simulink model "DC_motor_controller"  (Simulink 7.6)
settings: Solver=ode14x  StartTime=0.0  StopTime=10  FixedStep=2e-5  RelTol=1e-3
InitFcn:
  | Ts=2e-5;
  | Kp=200;
  | Ki=300;
  | Acceler_max=250;
  | 
  | Kpi=10;
  | Kii=50;
StopFcn:
  | clc
  | close all
  | clear all
  | 
  | load Vit_Ia.mat
  | subplot 211
  | plot(x(1,:),x(3,:))
  | grid
  | axis([0 10 0 450])
  | title('courant Ia')
  | xlabel('temps')
  | 
  | subplot 212
  | plot(x(1,:),x(2,:),x(1,:),x(3,:))
  | title('Consigne et vitesse de rotation')
  | axis([0 10 0 450])
  | grid
  | xlabel('temps')
  | 
  | delete *.mat
undefined symbols (not defined in the file or in its folder): sigbuilder_block
libraries: powerlib x2, electricdrivelib x1

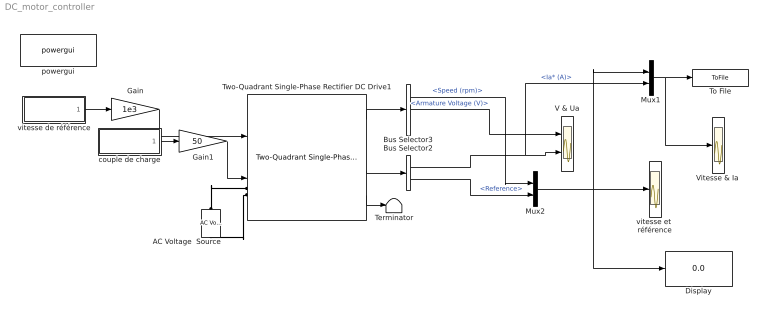
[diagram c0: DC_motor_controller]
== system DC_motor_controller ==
  AC Voltage  Source : powerlib/Electrical Sources/AC Voltage Source  DialogController=POWERSYS.PowerSysDialog  SystemSampleTime=-1  Amplitude=220  Phase=0  Frequency=60  SampleTime=0  Measurements=None
  Bus Selector2 : BusSelector  OutputSignals=Ia* (A),Reference
  Bus Selector3 : BusSelector  OutputSignals=Speed (rpm),Armature Voltage (V),Armature current ia (A)
  Display : Display
  Gain : Gain  Gain=1e3
  Gain1 : Gain  Gain=50
  Mux1 : Mux  Inputs=2
  Mux2 : Mux  Inputs=2
  Terminator : Terminator
  To File : ToFile  Filename=Vit_Ia  MatrixName=x
  Two-Quadrant Single-Phase Rectifier DC Drive1 : electricdrivelib/DC drives/Two-Quadrant Single-Phase Rectifier DC Drive  SystemSampleTime=-1  showMaskWarnings=on  AverageValue=off  MechanicalLoad=Torque Tm  driveType=DC1
  V & Ua : Scope  NumInputPorts=2
  "Vitesse & Ia " : Scope
  couple de charge : Subsystem  Tag=STV Subsys  LoadFcn=sigbuilder_block('load',[174.75 28.5 550.5 399.75 ]);  StartFcn=sigbuilder_block('start');  StopFcn=sigbuilder_block('stop');  ClipboardFcn=sigbuilder_block('clipboard');
  powergui : powerlib/powergui  Priority=2  SystemSampleTime=-1  SimulationMode=Discrete  SampleTime=2e-5  frequency=60  SPID=off  DisableSnubberDevices=off  DisableRonSwitches=off  DisableVfSwitches=off  SwTol=0  Interpol=off  frequencyindice=0  echomessages=off  HookPort=off  DisplayEquations=off  FunctionMessages=off  EnableUseOfTLC=off  x0status=blocks  RestoreLinks=warning  ResistiveCurrentMeasurement=off  Frange=[0:2:500]  Ylog=off  Xlog=on  ShowGrid=off  save=off  variable=ZData  ZoomFFT=on  StartTime=0.0  cycles=1  DisplayStyle=1  fundamental=60  FreqAxis=off  MaxFrequency=1000  frequencyindicesteady=1  RmsSteady=1  display=off  Ts=0  methode=off
  vitesse de référence : Subsystem  Tag=STV Subsys  LoadFcn=sigbuilder_block('load');  StartFcn=sigbuilder_block('start');  StopFcn=sigbuilder_block('stop');  ClipboardFcn=sigbuilder_block('clipboard');
  vitesse et  référence : Scope
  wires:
  Gain/1 -> Two-Quadrant Single-Phase Rectifier DC Drive1/1
  Two-Quadrant Single-Phase Rectifier DC Drive1/1 -> Bus Selector3/1
  Two-Quadrant Single-Phase Rectifier DC Drive1/3 -> Bus Selector2/1
  Two-Quadrant Single-Phase Rectifier DC Drive1/4 -> Terminator/1
  Bus Selector3/2 -> V & Ua/1  "<Armature Voltage (V)>"
  Mux2/1 -> Display/1, vitesse et  référence/1, Mux1/1
  Bus Selector2/2 -> Mux2/2  "<Reference>"
  Bus Selector3/1 -> Mux2/1  "<Speed (rpm)>"
  vitesse de référence/1(Signal 1) -> Gain/1
  Bus Selector2/1 -> V & Ua/2, Mux1/2  "<Ia* (A)>"
  Mux1/1 -> To File/1, "Vitesse & Ia "/1
  couple de charge/1(Signal 1) -> Gain1/1
  Gain1/1 -> Two-Quadrant Single-Phase Rectifier DC Drive1/2
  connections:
  AC Voltage  Source/RConn1 -- Two-Quadrant Single-Phase Rectifier DC Drive1/LConn1
  Two-Quadrant Single-Phase Rectifier DC Drive1/LConn2 -- AC Voltage  Source/LConn1

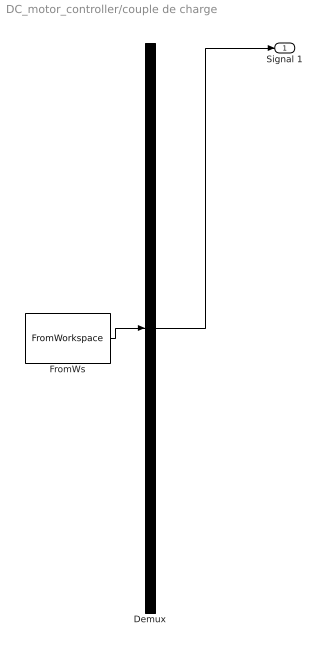
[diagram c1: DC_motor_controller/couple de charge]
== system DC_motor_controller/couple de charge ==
  Demux : Demux  Tag=STV Demux  Outputs=1
  FromWs : FromWorkspace  Tag=STV FromWs  VariableName=tuvar  SampleTime=0  SigBuilderData=DataTag1  VnvData=DataTag2
  Signal 1 : Outport  Tag=STV Outport
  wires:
  Demux/1 -> Signal 1/1
  FromWs/1 -> Demux/1

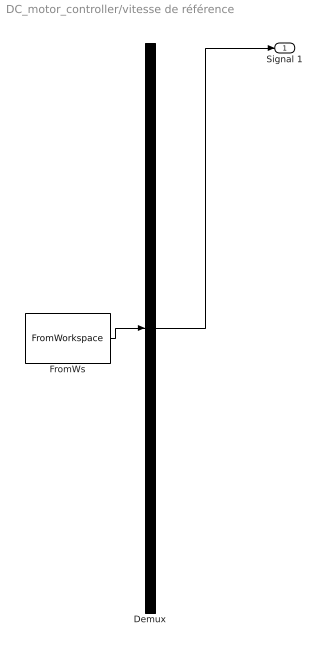
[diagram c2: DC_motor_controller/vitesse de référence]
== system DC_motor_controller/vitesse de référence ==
  Demux : Demux  Tag=STV Demux  Outputs=1
  FromWs : FromWorkspace  Tag=STV FromWs  VariableName=tuvar  SampleTime=0  SigBuilderData=DataTag4  VnvData=DataTag5
  Signal 1 : Outport  Tag=STV Outport
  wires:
  Demux/1 -> Signal 1/1
  FromWs/1 -> Demux/1
